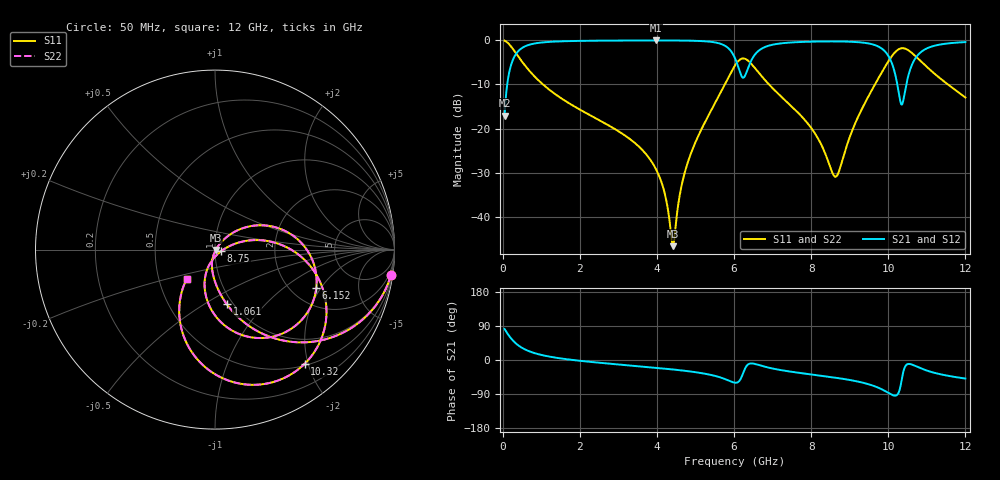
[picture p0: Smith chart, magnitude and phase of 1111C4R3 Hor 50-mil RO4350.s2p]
# GHz S MA R 50
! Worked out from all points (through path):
!   11951 points, 50 MHz to 12 GHz, reference 50 ohm
!   highest |S21| = -0.03 dB at 3.969 GHz (marker M1); lowest = -17.0 dB at 50 MHz (marker M2)
!   group delay of S21, straight-line fit = 17.5 ps
!   lowest |S11| = -46.6 dB at 4.416 GHz (marker M3), VSWR 1.01, Z = 50.4 - j0.224 ohm
!   |S11| at or under -10 dB: 1.045 GHz to 5.759 GHz (4.714 GHz wide, 139 % of centre); 6.906 GHz to 9.655 GHz (2.748 GHz wide, 33.2 % of centre); 11.55 GHz to end of sweep
!   |S22| runs from -46.6 to -0.1 dB; largest |S21 - S12| = 0
!   S11 on the Smith chart (normalised r, x): 50 MHz: 1, -14; 1.061 GHz: 0.94, -0.63; 6.152 GHz: 2.70, -1.82; 8.75 GHz: 1.07, -0.02; 10.32 GHz: 0.53, -1.94; 12 GHz: 0.70, -0.24
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0.05  0.9901 -8.4  0.1406 81.6  0.1406 81.6  0.9901 -8.4
0.328  0.7311 -44.9  0.6817 45.1  0.6817 45.1  0.7311 -44.9
1.061  0.3118 -77.8  0.9491 12.0  0.9491 12.0  0.3118 -77.8
2.042  0.1604 -92.0  0.9855 -2.5  0.9855 -2.5  0.1604 -92.0
3.969  0.03513 -105.6  0.9961 -20.6  0.9961 -20.6  0.03513 -105.6
4.034  0.03066 -105.1  0.9961 -21.2  0.9961 -21.2  0.03066 -105.1
4.416  0.004657 -28.5  0.9951 -25.0  0.9951 -25.0  0.004657 -28.5
4.852  0.04818 49.9  0.9902 -30.1  0.9902 -30.1  0.04818 49.9
5.548  0.2102 36.1  0.9387 -43.0  0.9387 -43.0  0.2102 36.1
6.025  0.5189 -1.3  0.6263 -60.0  0.6263 -60.0  0.5189 -1.3
6.152  0.6036 -20.7  0.4364 -53.2  0.4364 -53.2  0.6036 -20.7
6.391  0.5742 -58.4  0.5205 -10.2  0.5205 -10.2  0.5742 -58.4
6.772  0.367 -89.9  0.8284 -17.0  0.8284 -17.0  0.367 -89.9
8.017  0.09951 -111.2  0.9657 -38.3  0.9657 -38.3  0.09951 -111.2
8.585  0.02958 -63.4  0.9713 -46.0  0.9713 -46.0  0.02958 -63.4
8.75  0.03583 -13.4  0.97 -48.5  0.97 -48.5  0.03583 -13.4
9.628  0.3013 9.0  0.8903 -68.6  0.8903 -68.6  0.3013 9.0
10.009  0.5839 -14.1  0.6585 -87.2  0.6585 -87.2  0.5839 -14.1
10.323  0.8089 -51.9  0.1954 -66.1  0.1954 -66.1  0.8089 -51.9
10.525  0.7693 -77.5  0.4052 -10.4  0.4052 -10.4  0.7693 -77.5
10.866  0.5661 -104.7  0.7466 -23.0  0.7466 -23.0  0.5661 -104.7
12  0.225 -134.1  0.9548 -49.0  0.9548 -49.0  0.225 -134.1
